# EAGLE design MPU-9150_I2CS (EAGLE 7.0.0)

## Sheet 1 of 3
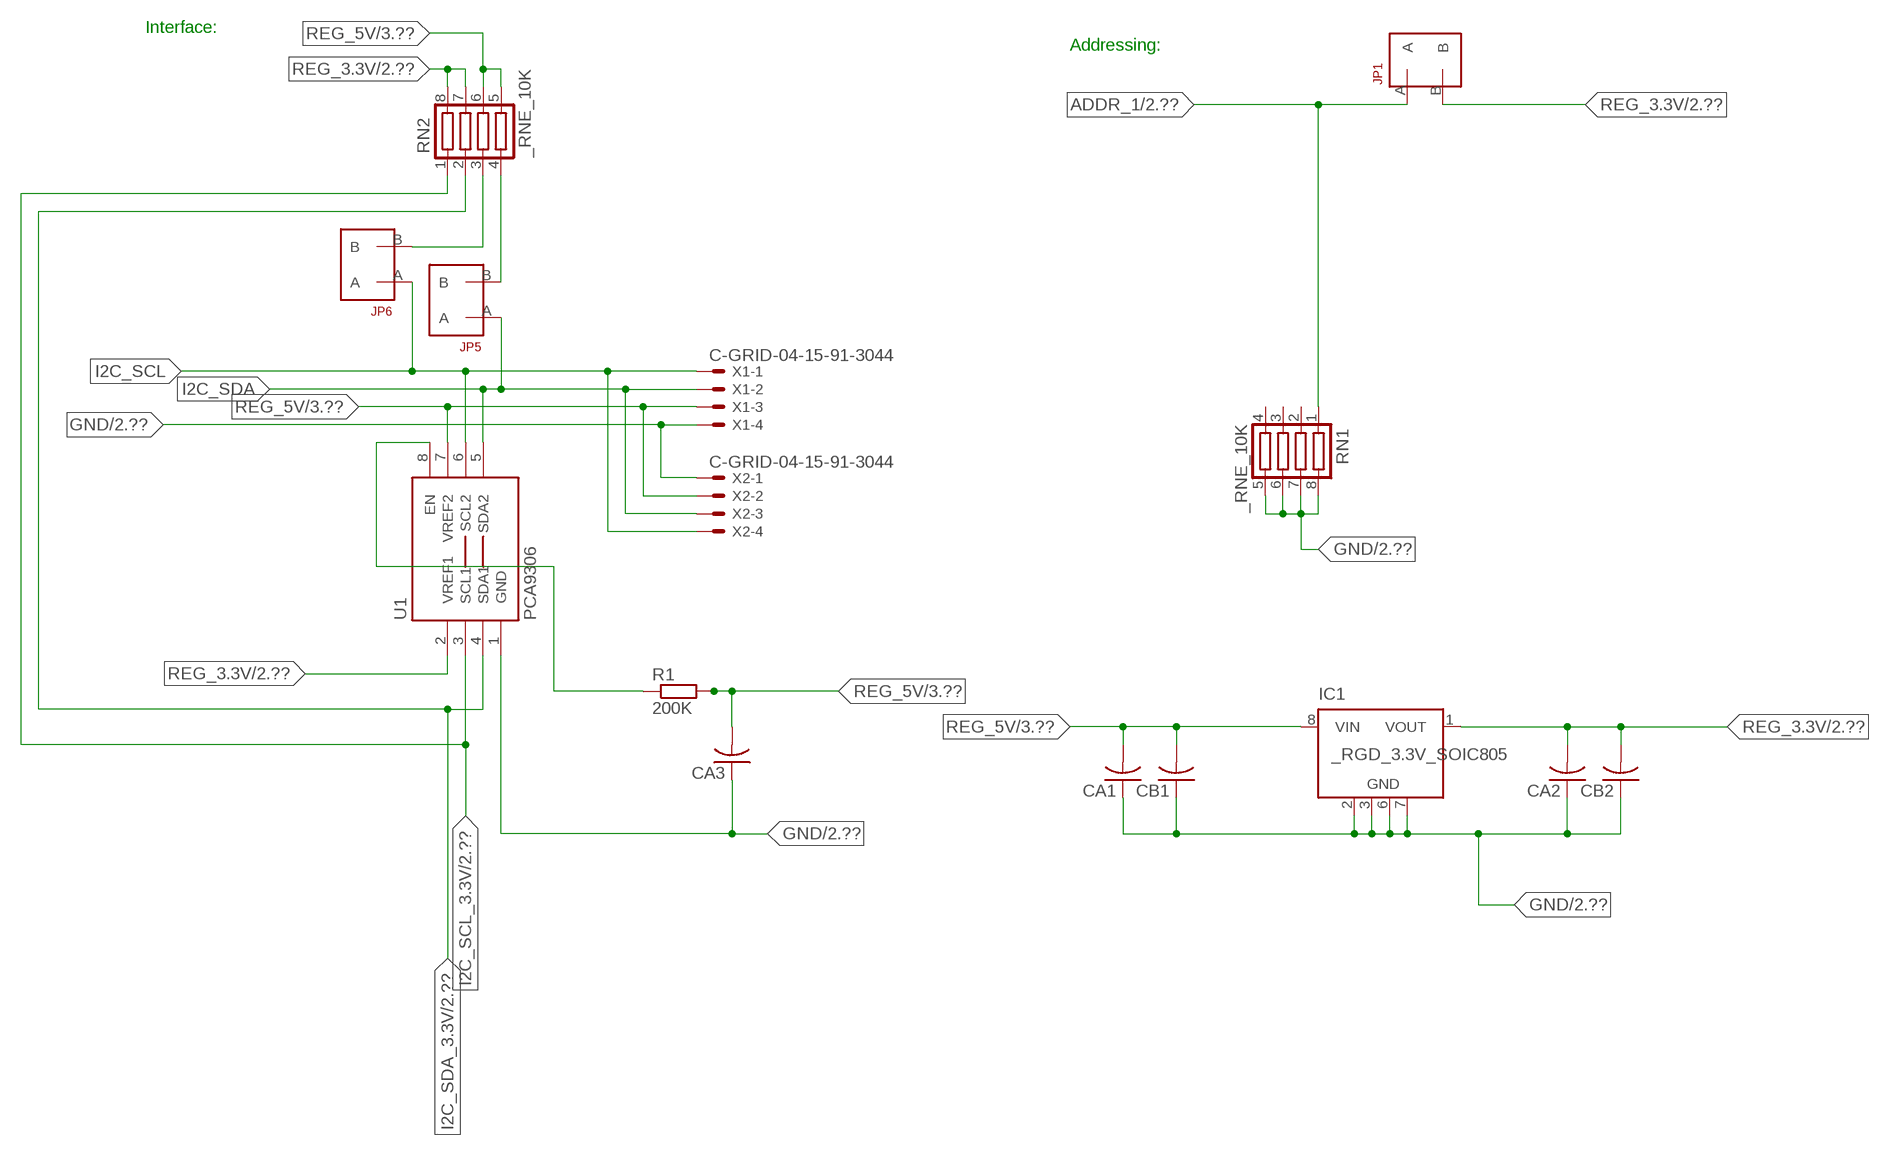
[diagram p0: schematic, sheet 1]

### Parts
CA1  CC1206KRX7R9BB104  [.1UF]
CA2  CC1206KRX7R9BB104  [.1UF]
CA3  CC1206KRX7R9BB104  [.1UF]
CB1  TMK316F106ZL-TC1206K  [TMK316F106ZL-T]
CB2  TMK316F106ZL-TC1206K  [TMK316F106ZL-T]
IC1  _RGD_3.3V_SOIC805  [_RGC_3.3V_SOIC8]
JP1  JUMPER_1X2_2MM  [JUMPER_1X2_2MM]
JP5  JUMPER_1X2_2MM  [JUMPER_1X2_2MM]
JP6  JUMPER_1X2_2MM  [JUMPER_1X2_2MM]
R1  200K  RESISTOR_SMT-0603  [R603]
RN1  _RNE_10K  [RNE]
RN2  _RNE_10K  [RNE]
U1  PCA9306  PCA9306_NCD  [PSOP-8]
X1  C-GRID-04-15-91-3044  [15-91-04]
X2  C-GRID-04-15-91-3044  [15-91-04]

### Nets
ADDR_1: JP1.A RN1.1 ; also sheet 2
GND: CA1.1 CA2.1 CA3.1 CB1.1 CB2.1 IC1.2(GND) IC1.3(GND) IC1.6(GND) IC1.7(GND) RN1.5 RN1.6 RN1.7 RN1.8 U1.1(GND) X1.4 X2.1 ; also sheet 2,3
I2C_SCL: JP6.A U1.6(SCL2) X1.1 X2.4
I2C_SCL_3.3V: RN2.1 U1.3(SCL1) ; also sheet 2
I2C_SDA: JP5.A U1.5(SDA2) X1.2 X2.3
I2C_SDA_3.3V: RN2.2 U1.4(SDA1) ; also sheet 2
N$1: JP6.B RN2.3
N$2: JP5.B RN2.4
N$3: R1.1 U1.8(EN)
REG_3.3V: CA2.2 CB2.2 IC1.1(VOUT) JP1.B RN2.7 RN2.8 U1.2(VREF1) ; also sheet 2
REG_5V: CA1.2 CA3.2 CB1.2 IC1.8(VIN) R1.2 RN2.5 RN2.6 U1.7(VREF2) X1.3 X2.2 ; also sheet 3
Unconnected: IC1.4(NC) IC1.5(NC) RN1.2 RN1.3 RN1.4

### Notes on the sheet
- Interface:
- Addressing:

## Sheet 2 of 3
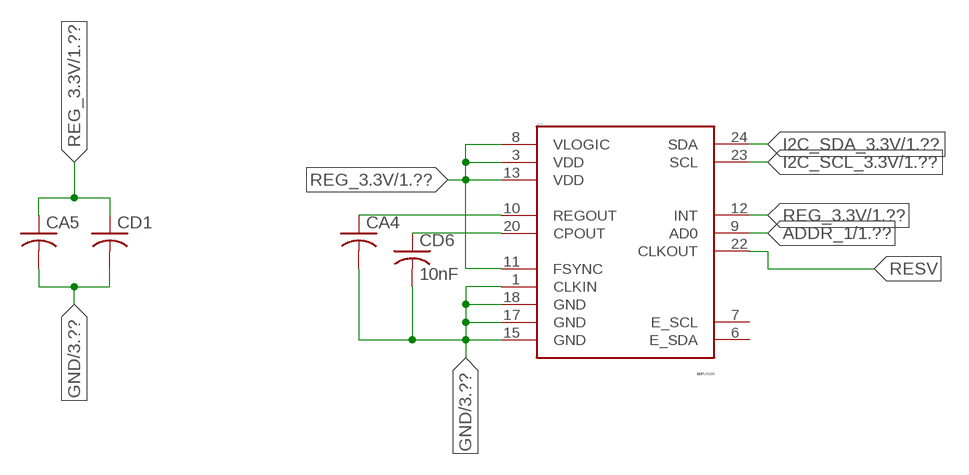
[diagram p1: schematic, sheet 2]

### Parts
CA4  CC1206KRX7R9BB104  [.1UF]
CA5  CC1206KRX7R9BB104  [.1UF]
CD1  CC1206KRX7R9BB103C1206K  [CC1206KRX7R9BB103]
CD6  10nF  _CD_10NF_50VC1206K  [_CD_10NF_50V]
IC2  MPU9150  SPARKFUN-SENSORS_MPU-9150QFN-24-NP  [SPARKFUN-SENSORS_QFN-24-NP]

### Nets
ADDR_1: IC2.9(AD0) ; also sheet 1
GND: CA4.2 CA5.2 CD1.2 CD6.2 IC2.1(CLKIN) IC2.15(GND) IC2.17(GND) IC2.18(GND) ; also sheet 1,3
I2C_SCL_3.3V: IC2.23(SCL) ; also sheet 1
I2C_SDA_3.3V: IC2.24(SDA) ; also sheet 1
N$14: CA4.1 IC2.10(REGOUT)
N$15: CD6.1 IC2.20(CPOUT)
REG_3.3V: CA5.1 CD1.1 IC2.3(VDD) IC2.8(VLOGIC) IC2.11(FSYNC) IC2.12(INT) IC2.13(VDD) ; also sheet 1
RESV: IC2.22(CLKOUT)
Unconnected: IC2.6(E_SDA) IC2.7(E_SCL)

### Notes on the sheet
- IC2

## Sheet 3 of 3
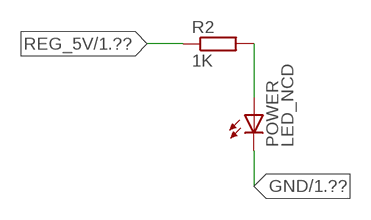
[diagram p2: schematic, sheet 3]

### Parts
POWER  LED_NCD  [CHIPLED_0603]
R2  1K  RESISTOR_SMT-0402  [R402]

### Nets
GND: POWER.C ; also sheet 1,2
N$4: POWER.A R2.2
REG_5V: R2.1 ; also sheet 1

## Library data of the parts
CA1-CA3 = NCD_ULTIMATE_LIBRARY:CC1206KRX7R9BB104: Capacitor CA .1uF 50V SMT C1206K CC1206KRX7R9BB104
CA4 CA5 = NCD_ULTIMATE_LIBRARY (1):CC1206KRX7R9BB104: Capacitor CA .1uF 50V SMT C1206K CC1206KRX7R9BB104
CB1 CB2 = NCD_ULTIMATE_LIBRARY:TMK316F106ZL-T: Capacitor CB 10uF SMT 1206 TMK316F106ZL-T
CD1 = NCD_ULTIMATE_LIBRARY (1):CC1206KRX7R9BB103: Capacitor CD .01uF SMT CC1206KRX7R9BB103 1206
CD6 = NCD_ULTIMATE_LIBRARY:_CD_10NF_50V: Capacitor 10nF SMT
IC1 = NCD_ULTIMATE_LIBRARY:_RGD_3.3V_SOIC8: Regulator Linear 3.3V Chip Positive VOLTAGE REGULATOR Digikey 497-1199-2-ND/L78L33ACD13TR
IC2 = NCD_ULTIMATE_KAMNA:SPARKFUN-SENSORS_MPU-9150: 9DOF (3mag, 3accel, 3rotat). I2C interface.
JP1 JP5 JP6 = NCD_ULTIMATE_CONNECTORS:JUMPER_1X2_2MM
POWER = NCD_ULTIMATE_LIBRARY:LED_NCD: LED Digikey 754-1132-2-ND/APT2012SRCPRV
R1 R2 = NCD_ULTIMATE_LIBRARY:RESISTOR_SMT: NCD Resistor
RN1 RN2 = NCD_ULTIMATE_LIBRARY:_RNE_10K: Resistor Array RNE SMT 10K x 4 Single Resistor Source: http://www.ctscorp.com/components/Datasheets/CTSChipArrayDs.pdf Digikey 742C083103JPTR-ND/742C083103JP; OC_FARNELL: unknown; OC_NEWARK: unknown
U1 = NCD_ULTIMATE_LIBRARY:PCA9306_NCD: NCD Bidirectional I2C level shifter. NOT compatible with all available part number pinout schemes- DOUBLE CHECK!!!; PROD_ID: IC-10023
X1 X2 = NCD_ULTIMATE_CONNECTORS:C-GRID-04: CONNECTOR 4-Pos I2C wire to board 2.54 mm (0.100") pitch header Digikey WM1342-ND/0015912045; OC_FARNELL: unknown; OC_NEWARK: unknown

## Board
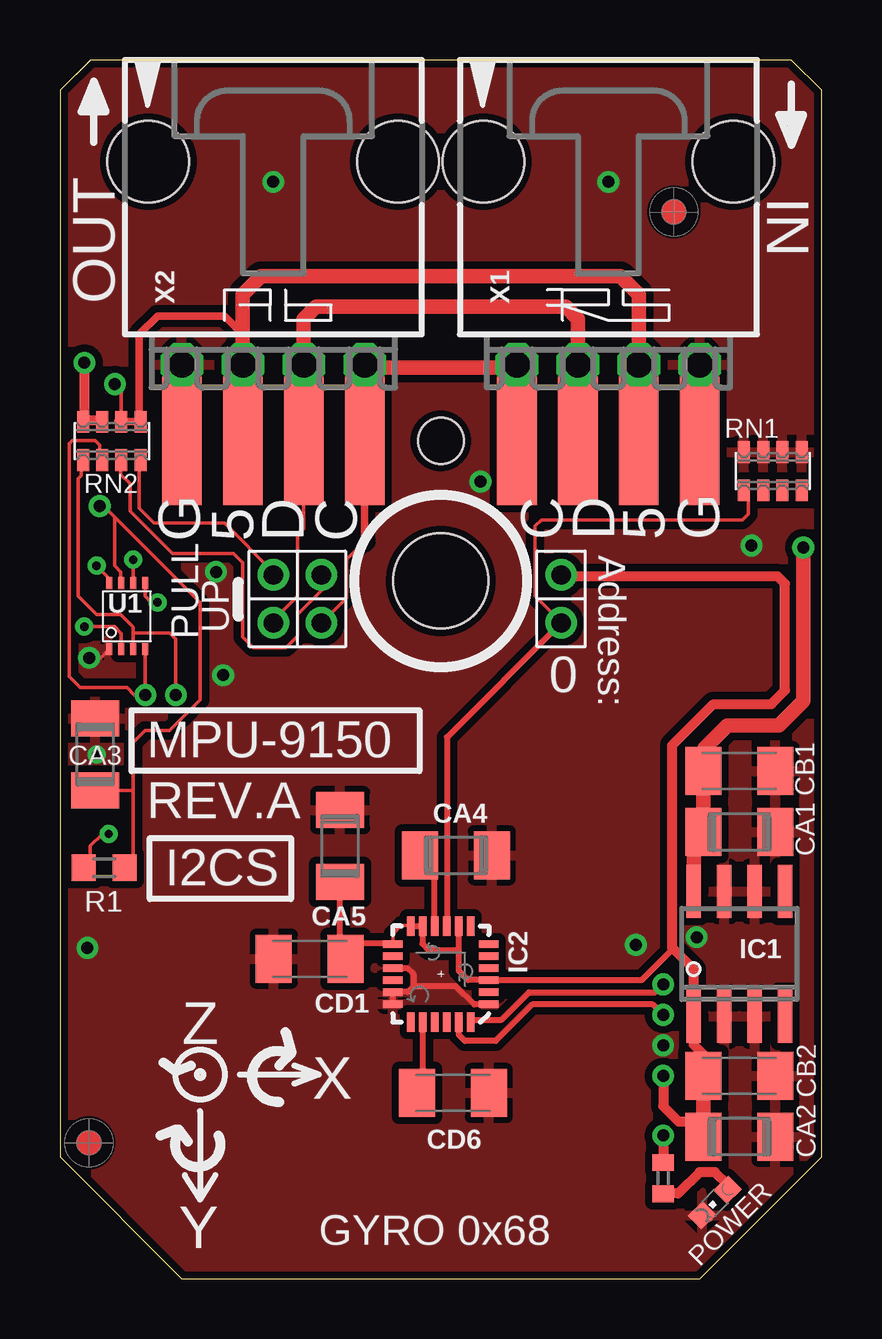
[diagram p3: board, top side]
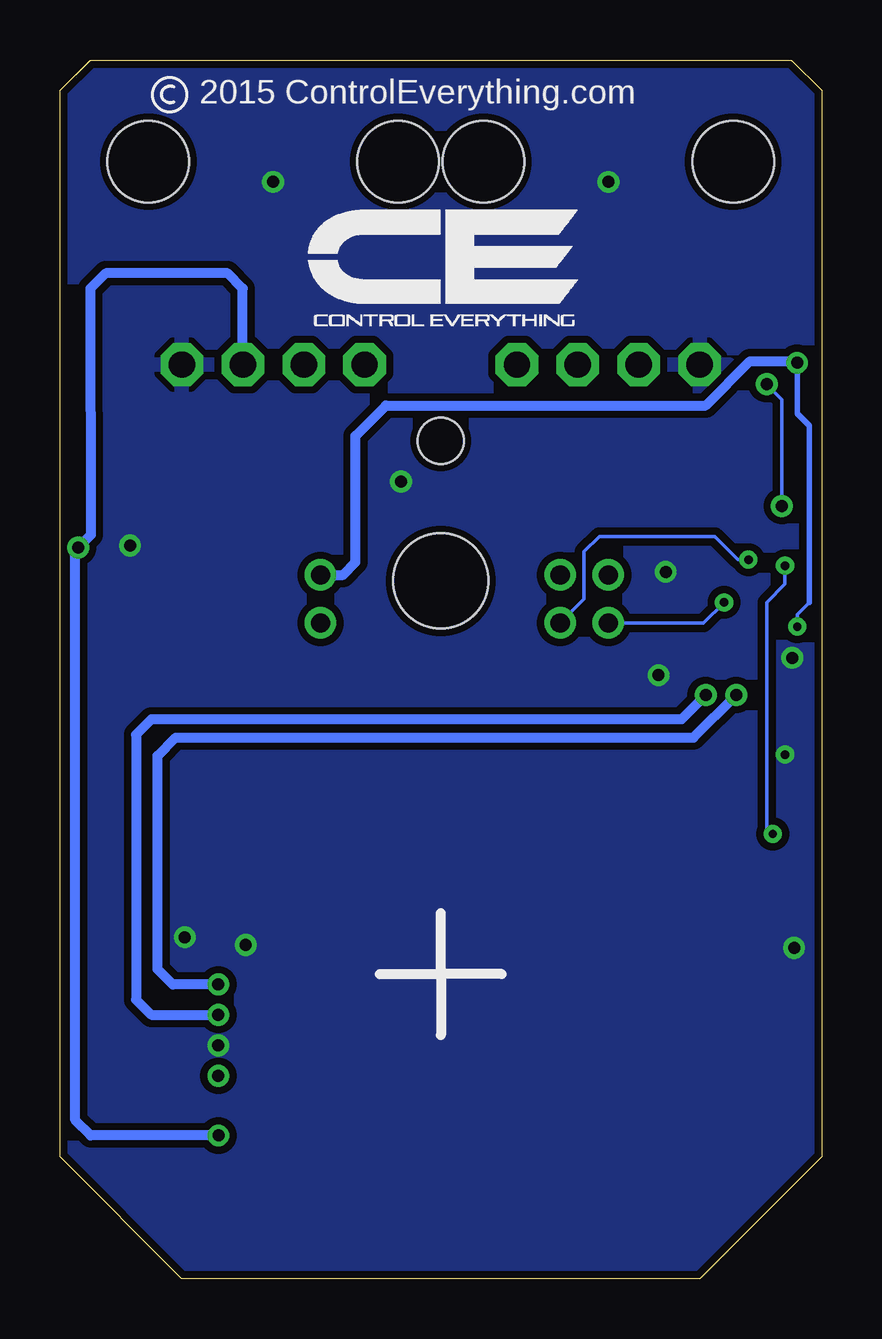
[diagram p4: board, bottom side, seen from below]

Size 31.75 x 50.8 mm. Coordinates in mm from the lower left corner, seen from the top.
Outline: 31.75,5.08 31.75,49.53 30.48,50.8 1.27,50.8 0,49.53 0,5.08 5.08,0 26.67,0 31.75,5.08
Outline: 31.75,5.08 31.75,49.53 30.48,50.8 1.27,50.8 0,49.53 0,5.08 5.08,0 26.67,0 31.75,5.08
Copper layers (1*16): Top 0.035mm / dielectric 1.5mm / Bottom 0.035mm
Design rules "default": minimum track width 5mil, minimum drill 24mil, track to track 5mil, track to pad 5mil, pad to pad 5mil, via to via 5mil, smd to smd 5mil, copper to edge 10mil, drill to drill 8mil, minimum pad ring 10mil, minimum via ring 8mil, stop-mask expansion 2mil, vias tented up to drill 0mil, thermal gap 10mil
Holes 3.96 mm at 15.88,29.08
Holes 1.91 mm at 15.88,34.93

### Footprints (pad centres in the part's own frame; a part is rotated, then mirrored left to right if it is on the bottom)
.1UF = smd 1.5 x 2: 1 -1.5,0; 2 1.5,0
TMK316F106ZL-T = smd 1.5 x 2: 1 -1.5,0; 2 1.5,0
CC1206KRX7R9BB103 = smd 1.5 x 2: 1 -1.5,0; 2 1.5,0
_CD_10NF_50V = smd 1.5 x 2: 1 -1.5,0; 2 1.5,0
_RGC_3.3V_SOIC8 = smd 0.6 x 2.2: 1 -1.905,-2.6; 2 -0.635,-2.6; 3 0.635,-2.6; 4 1.905,-2.6; 5 1.905,2.6; 6 0.635,2.6; 7 -0.635,2.6; 8 -1.905,2.6
SPARKFUN-SENSORS_QFN-24-NP = smd 0.8 x 0.3: 1 -2,1.25; 2 -2,0.75; 3 -2,0.25; 4 -2,-0.25; 5 -2,-0.75; 6 -2,-1.25; 13 2,-1.25; 14 2,-0.75; 15 2,-0.25; 16 2,0.25; 17 2,0.75; 18 2,1.25 | smd 0.3 x 0.8: 7 -1.25,-2; 8 -0.75,-2; 9 -0.25,-2; 10 0.25,-2; 11 0.75,-2; 12 1.25,-2; 19 1.25,2; 20 0.75,2; 21 0.25,2; 22 -0.25,2; 23 -0.75,2; 24 -1.25,2
JUMPER_1X2_2MM = drill 0.8: A 0,2; B 0,0
CHIPLED_0603 = smd 0.8 x 0.876: A 0,-0.75; C 0,0.75
R603 = smd 1 x 1.1: 1 -0.85,0; 2 0.85,0
R402 = smd 0.7 x 0.9: 1 -0.65,0; 2 0.65,0
RNE = smd 0.5 x 0.9: 1 -1.2,-0.8; 2 -0.4,-0.8; 3 0.4,-0.8; 4 1.2,-0.8; 5 1.2,0.8; 6 0.4,0.8; 7 -0.4,0.8; 8 -1.2,0.8
PSOP-8 = smd 0.25 x 0.5: 1 -0.73,-1.37; 2 -0.23,-1.37; 3 0.27,-1.37; 4 0.77,-1.37; 5 0.77,1.38; 6 0.27,1.38; 7 -0.23,1.38; 8 -0.73,1.38
15-91-04 = drill 1.1 pad 1.778 octagon: 1 -3.81,-7.62; 2 -1.27,-7.62; 3 1.27,-7.62; 4 3.81,-7.62 | smd 1.651 x 5.334: P1 -3.81,-10.795; P2 -1.27,-10.795; P3 1.27,-10.795; P4 3.81,-10.795 | hole 3.404: -5.207,0.838; 5.207,0.838

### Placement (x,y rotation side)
CA1  28.32,18.62 180 top
CA2  28.32,5.92 180 top
CA3  1.46,21.86 270 top
CA4  16.51,17.65 0 top
CA5  11.68,18.03 90 top
CB1  28.32,21.16 180 top
CB2  28.32,8.46 180 top
CD1  10.41,13.34 180 top
CD6  16.38,7.75 0 top
IC1  28.32,13.54 0 top
IC2  15.88,12.7 180 top
JP1  20.89,29.34 180 top
JP5  8.89,29.34 180 top
JP6  10.9,29.34 180 top
POWER  27.3,3.18 135 top
R1  1.84,17.13 0 top
R2  25.15,4.19 270 top
RN1  29.72,33.66 0 top
RN2  2.16,34.93 0 top
U1  2.79,27.61 0 top
U$5  [VISION_REF10]  1.21,5.66 90 top
U$28  [VISION_REF10]  25.59,44.46 90 top
X1  22.86,45.72 0 top
X2  8.89,45.72 0 top

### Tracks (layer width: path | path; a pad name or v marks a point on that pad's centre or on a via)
ADDR_1
  Top 0.152: JP1.A 20.89,27.37 19.81,28.45 19.81,31.37 20.07,31.62 28.45,31.62 28.7,31.88 28.7,32.78 RN1.1
  Top 0.254: JP1.A 16.12,22.57 IC2.9
GND  (via drill 0.35, 0.5)
  Top 0.152: CA3.1 1.52,23.42 1.52,23.62 | U1.1 1.7,25.88 v1.22,25.88
  Top 0.254: IC2.18 IC2.17 14.49,11.95 14.73,12.19 | IC2.15 14.48,12.95 14.73,12.7 14.73,12.19 | IC2.1 17.86,11.43 17.27,11.43 16.51,12.19 14.73,12.19
  other vias: 8.89,45.72 22.86,45.72 25.15,9.73 6.8,25.16 17.53,33.22 26.55,14.24 1.15,13.79 6.5,29.46 1.52,21.84 24.01,13.92 28.83,30.56
  pour Top (isolate 0.305): -1.27,0 -1.27,50.8 33.02,50.8 33.02,0
  pour Bottom (isolate 0.305): -5.08,0 -5.08,50.8 35.56,50.8 35.56,0
I2C_SCL  (via drill 0.35)
  Top 0.152: 12.7,30.73 11.94,29.97 11.94,28.38 JP6.A | v3.05,29.97 3.06,29.96 U1.6
  Top 0.305: 12.7,30.73 X2.4
  Top 0.406: X2.4 12.7,37.97 | 19.05,37.97 X1.1
  Top 0.61: 12.7,37.97 19.05,37.97
  Bottom 0.152: JP6.A 9.91,28.33 9.91,30.3 9.27,30.94 4.45,30.94 3.48,29.97 v3.05,29.97
I2C_SCL_3.3V  (via drill 0.5)
  Top 0.152: RN2.1 0.89,34.07 0.89,33.48 0.77,33.35 0.77,29.1 0.76,29.09 0.76,28.45 1.52,27.69 2.54,27.69 3.06,27.17 3.06,26.92 | 3.06,26.92 U1.3 | v4.83,24.33 v4.83,24.34 4.83,26.67 4.57,26.92 3.06,26.92
  Top 0.254: IC2.23 16.62,10.17 16.89,9.91 18.16,9.91 19.68,11.43 24.72,11.43 v25.15,11
  Bottom 0.406: v4.83,24.33 5.84,23.32 27.94,23.32 28.58,22.68 28.58,11.63 27.94,11 v25.15,11
I2C_SDA  (via drill 0.35)
  Top 0.152: JP5.A 8.89,27.44 9.91,28.45 9.91,30.99 10.16,31.24 10.16,34.92 X2.3 | U1.5 3.56,28.45 3.81,28.19 v4.06,28.19
  Top 0.305: 10.35,34.73 X2.3
  Top 0.61: X2.3 10.16,40.01 10.67,40.51 21.09,40.51 21.59,40.01 X1.2
  Bottom 0.152: v4.06,28.19 4.92,27.34 JP5.A
I2C_SDA_3.3V  (via drill 0.5)
  Top 0.152: RN2.2 1.65,34.14 1.65,34.75 1.46,34.94 0.51,34.94 0.38,34.81 0.38,26.37 0.38,26.36 0.38,25.1 0.84,24.64 2.79,24.64 3.1,24.33 v3.56,24.33 v3.56,24.34 U1.4
  Top 0.254: IC2.24 17.22,10.8 18.41,10.8 19.56,11.94 24.82,11.94 v25.15,12.27
  Bottom 0.406: v25.15,12.27 27.05,12.27 27.69,12.9 27.69,21.79 26.93,22.56 5.34,22.56 v3.56,24.33
N$1
  Top 0.152: JP6.B 10.92,29.31 10.92,28.7 9.91,27.69 9.91,26.8 9.42,26.31 8.06,26.31 7.62,26.75 7.62,29.84 7.24,30.23 4.7,30.23 2.92,32 2.92,33.15 2.54,33.53 2.54,34.1 RN2.3
  Top 0.305: 2.54,34.02 RN2.3
N$2
  Top 0.152: JP5.B 8.89,29.46 6.86,31.5 3.94,31.5 3.3,32.13 3.3,34.07 RN2.4
  Top 0.305: 3.37,33.88 RN2.4
N$3  (via drill 0.35)
  Top 0.152: R1.1 1.27,17.41 1.27,18.03 1.78,18.54 v2.03,18.54 | v1.52,29.72 2.06,29.18 U1.8
  Bottom 0.152: v2.03,18.54 2.29,18.8 2.29,28.19 1.52,28.96 v1.52,29.72
N$4
  Top 0.406: POWER.A 27.84,3.92 27.3,4.45 26.67,4.45 25.78,3.56 25.16,3.56 R2.2
N$14
  Top 0.254: IC2.10 15.62,17.27 15.24,17.65 CA4.1
N$15
  Top 0.254: CD6.1 15.12,7.99 IC2.20
REG_3.3V  (via drill 0.35, 0.5)
  Top 0.152: v1.02,27.18 2.29,27.18 2.56,26.9 U1.2 | IC2.12 14.59,14.73 14.22,14.73 13.88,14.38 IC2.13
  Top 0.254: IC2.13 13.86,13.97 12.19,13.97 11.91,13.69 CD1.1 11.68,13.57 CA5.1 | IC2.12 IC2.11 15.11,14.69 15.11,13.97 15.37,13.72 16.62,13.72 | 16.62,13.72 IC2.8 | 25.53,13.79 25.53,13.72 24.26,12.45 IC2.3 17.02,12.45 16.62,12.84 16.62,13.72
  Top 0.406: CB2.2 26.82,9.35 26.42,9.75 26.42,10.36 | v25.15,8.46 25.15,7.19 25.78,6.55 26.82,6.55 | IC1.1 26.42,12.9 25.53,13.79 25.53,22.24 27.24,23.95 29.66,23.95 30.23,24.52 30.23,28.97 29.91,29.29 20.95,29.29 JP1.B | 26.52,5.62 CA2.2 | v1.02,38.18 1.02,35.78 | 1.02,35.78 RN2.8 | 1.02,35.78 1.71,35.78 RN2.7
  Top 0.61: CB2.2 26.82,6.55 CA2.2 | 26.42,10.36 IC1.1
  Bottom 0.152: 0.51,28.19 1.02,27.69 v1.02,27.18
  Bottom 0.229: 0.51,28.19 0.51,35.56 1.02,36.07 v1.02,38.18
  Bottom 0.406: v1.02,38.18 1.08,38.24 2.99,38.24 4.83,36.4 18.16,36.4 19.43,35.13 19.43,29.87 19.94,29.34 JP1.B
REG_5V  (via drill 0.5)
  Top 0.152: RN2.6 2.56,37.01 v2.29,37.29 | R1.2 3.05,17.49 3.05,20.36 | 3.05,20.36 3.05,22.35 3.56,22.86 4.57,22.86 5.84,24.13 5.84,28.19 2.29,31.75 | CA3.2 3.05,20.36 | 2.29,31.75 1.83,32.21 v1.65,32.21 | U1.7 2.54,29.01 2.54,29.46 2.29,29.72 2.29,31.75
  Top 0.305: 7.62,39.37 7.5,39.37 | 2.42,35.74 RN2.6 RN2.5 3.31,35.8 3.31,39.37 4.07,40.13 6.86,40.13 7.62,39.37 | X2.2 7.62,39.37
  Top 0.406: v25.15,5.97 R2.1
  Top 0.61: X2.2 7.62,41.02 8.38,41.78 23.37,41.78 24.13,41.02 X1.3 | IC1.8 26.42,18.21 CA1.2 CB1.2 26.86,21.2 26.86,22.11 27.82,23.06 29.98,23.06 30.99,24.08 v30.99,30.48
  Bottom 0.152: v1.65,32.21 1.65,36.65 v2.29,37.29
  Bottom 0.406: X1.3 24.13,41.28 24.77,41.91 29.84,41.91 30.48,41.27 30.47,31 v30.99,30.48 31.11,30.36 31.11,6.6 30.48,5.97 v25.15,5.97

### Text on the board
tNames: IN | OUT | G | 5 | D | C | C | D | 5 | G | Address: | PULL | UP | 0 | MPU-9150 | REV.A | I2CS | Z | X | Y | GYRO 0x68
bNames: 2015 ControlEverything.com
